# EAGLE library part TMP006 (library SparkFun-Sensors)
Infrared Temperature Sensor TMP006 3.3v to 5.0v Datasheet SparkFun Products SparkFun Infrared Temperature Breakout - TMP006 (SEN-11859)
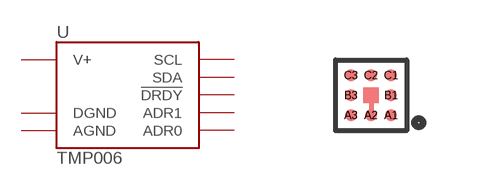
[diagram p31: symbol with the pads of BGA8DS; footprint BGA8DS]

Designator prefix -

## TMP006 (PROD_ID: IC-11632; VALUE: TMP006)  [BGA8DS]
A1  DGND
A2  AGND
A3  V+
B1  ADR1
B3  SCL
C1  ADR0
C2  !DRDY
C3  SDA

## Footprint BGA8DS (pad centres in mm)
smd 0.305 x 0.305: A1 0.5,-0.5; A2 0,-0.5; A3 -0.5,-0.5; B1 0.5,0; B3 -0.5,0; C1 0.5,0.5; C2 0,0.5; C3 -0.5,0.5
